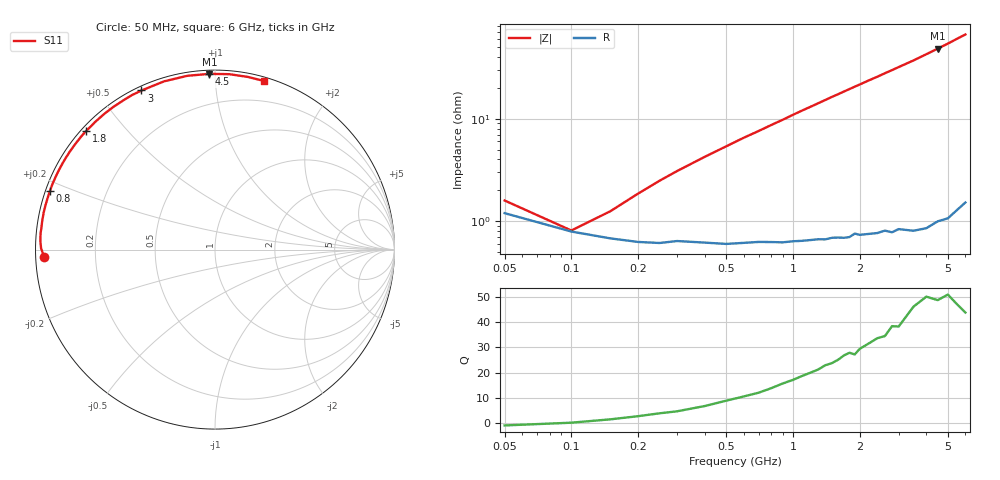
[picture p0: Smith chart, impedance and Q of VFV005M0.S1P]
! Infineon Technologies  Discrete & RF Semiconductors
! BBY 58-03
! Si Tuning Diode in SOD323
! VR =
! S-Parameters:  June  1999
# GHz  S  MA  R  50
!  f  S11
! GHz  MAG  ANG
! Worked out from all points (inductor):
!   34 points, 50 MHz to 6 GHz, reference 50 ohm
!   read as one part to ground: L = 1.6 nH near 250 MHz
!   highest Q = 50.1 at 4.5 GHz (marker M1), where L = 1.71 nH
!   S11 on the Smith chart (normalised r, x): 50 MHz: 0.02, -0.02; 800 MHz: 0.01, +0.17; 1.8 GHz: 0.01, +0.39; 3 GHz: 0.02, +0.64; 4.5 GHz: 0.02, +0.97; 6 GHz: 0.03, +1.33
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0.05  0.9533 -177.6
0.1  0.9689 179.6
0.15  0.9733 177.6
0.25  0.9759 174.5
0.4  0.9758 170.4
0.5  0.9766 167.8
0.6  0.9762 165.2
0.8  0.9761 160.3
0.9  0.9764 157.9
1  0.976 155.4
1.2  0.9759 150.7
1.4  0.976 146.1
1.5  0.9755 143.8
1.6  0.9757 141.7
1.7  0.9761 139.5
1.8  0.976 137.4
2  0.9756 133.3
2.2  0.9758 129.3
2.4  0.9761 125.6
2.6  0.9757 121.8
2.8  0.9774 118.3
3  0.9766 114.8
3.5  0.9795 106.8
4  0.9805 99.0
4.5  0.9797 91.8
5  0.9806 85.4
5.5  0.9794 79.2
6  0.9783 73.8
